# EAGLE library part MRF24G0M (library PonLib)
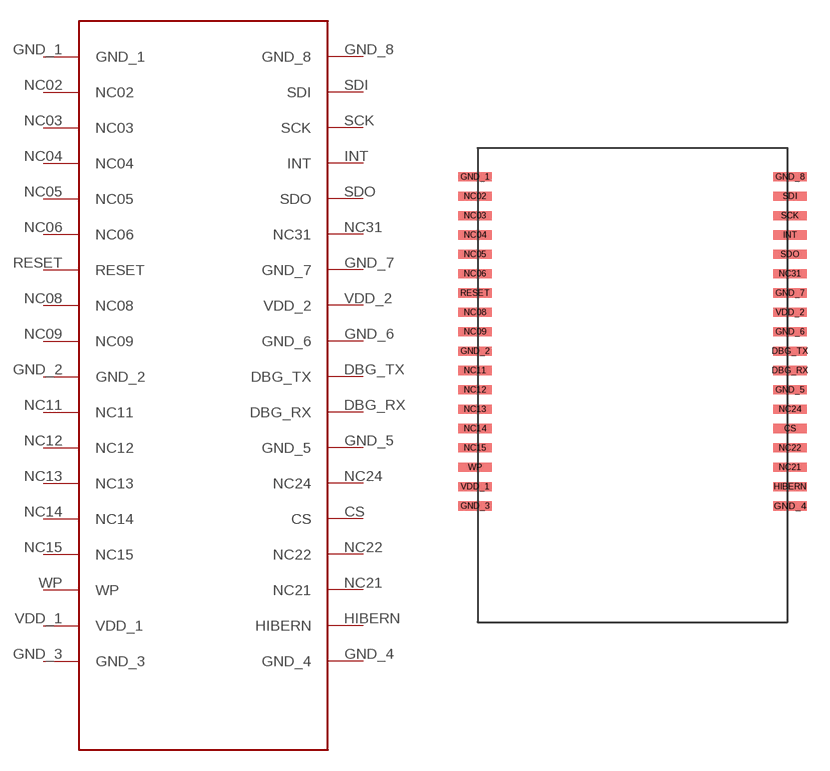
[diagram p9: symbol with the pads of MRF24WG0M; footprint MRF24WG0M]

Designator prefix -

## MRF24G0M  [MRF24WG0M]
CS  CS
DBG_RX  DBG_RX
DBG_TX  DBG_TX
GND_1  GND_1
GND_2  GND_2
GND_3  GND_3
GND_4  GND_4
GND_5  GND_5
GND_6  GND_6
GND_7  GND_7
GND_8  GND_8
HIBERN  HIBERN
INT  INT
NC02  NC02
NC03  NC03
NC04  NC04
NC05  NC05
NC06  NC06
NC08  NC08
NC09  NC09
NC11  NC11
NC12  NC12
NC13  NC13
NC14  NC14
NC15  NC15
NC21  NC21
NC22  NC22
NC24  NC24
NC31  NC31
RESET  RESET
SCK  SCK
SDI  SDI
SDO  SDO
VDD_1  VDD_1
VDD_2  VDD_2
WP  WP

## Footprint MRF24WG0M (pad centres in mm)
smd 2.2 x 0.6: CS 10.33,-5.715; DBG_RX 10.33,-1.905; DBG_TX 10.33,-0.635; GND_1 -10.33,10.795; GND_2 -10.33,-0.635; GND_3 -10.33,-10.795; GND_5 10.33,-3.175; GND_6 10.33,0.635; GND_7 10.33,3.175; GND_8 10.33,10.795; HIBERN 10.33,-9.525; INT 10.33,6.985; NC02 -10.33,9.525; NC03 -10.33,8.255; NC04 -10.33,6.985; NC05 -10.33,5.715; NC06 -10.33,4.445; NC08 -10.33,1.905; NC09 -10.33,0.635; NC11 -10.33,-1.905; NC12 -10.33,-3.175; NC13 -10.33,-4.445; NC14 -10.33,-5.715; NC15 -10.33,-6.985; NC21 10.33,-8.255; NC22 10.33,-6.985; NC24 10.33,-4.445; NC31 10.33,4.445; RESET -10.33,3.175; SCK 10.33,8.255; SDI 10.33,9.525; SDO 10.33,5.715; VDD_1 -10.33,-9.525; VDD_2 10.33,1.905; WP -10.33,-8.255
smd 2.2 x 0.635: GND_4 10.33,-10.795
